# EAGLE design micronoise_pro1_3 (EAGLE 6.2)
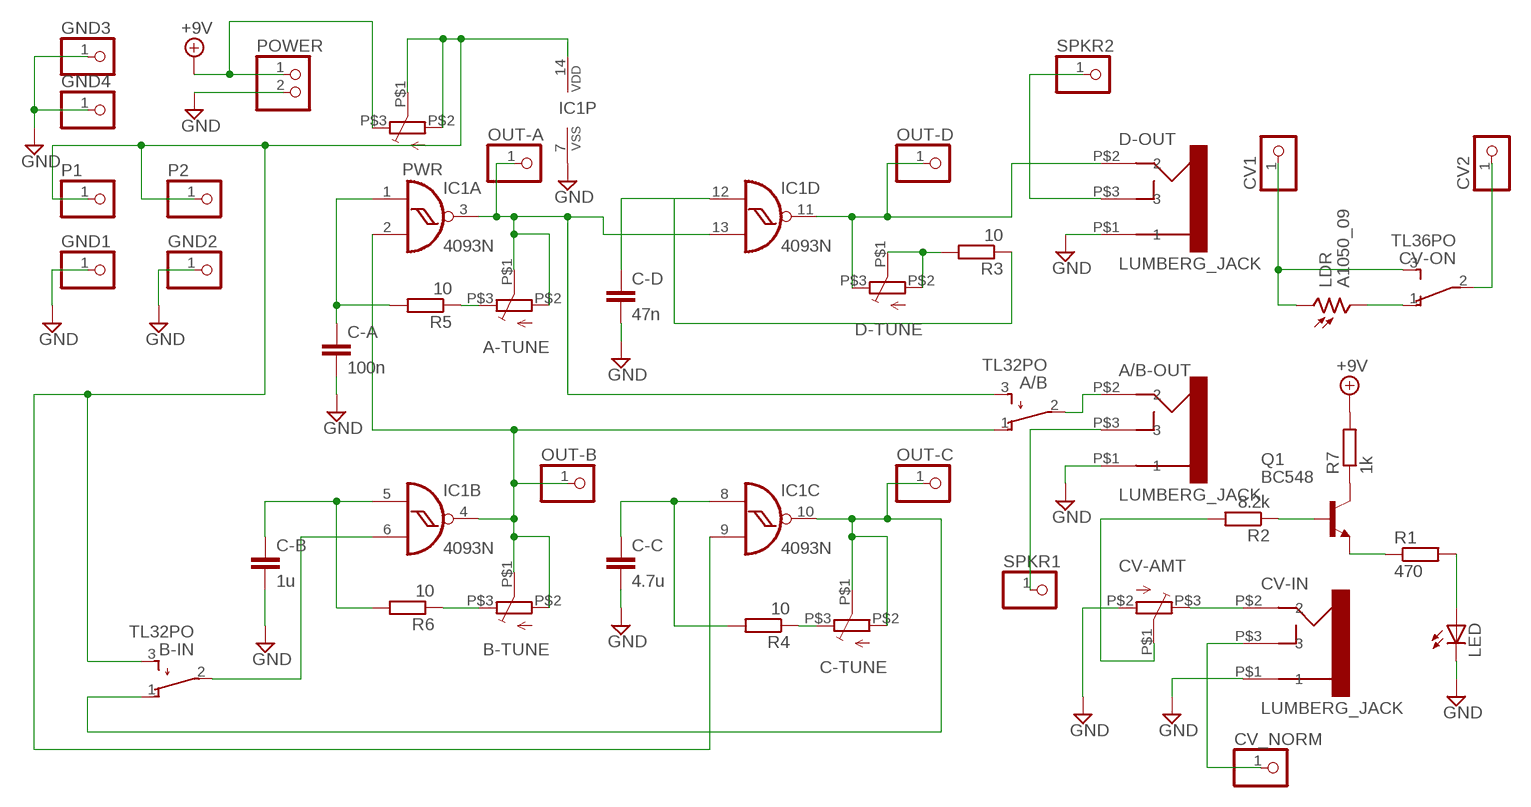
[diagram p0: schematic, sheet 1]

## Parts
A-TUNE  STR09K113  [STR09K113]
A/B  TL32PO  [TL3XPO]
A/B-OUT  LUMBERG_JACK  [JACK_CON]
B-IN  TL32PO  [TL3XPO]
B-TUNE  STR09K113  [STR09K113]
C-A  100n  C-EU050-035X075  [C050-035X075]
C-B  1u  C-EU050-035X075  [C050-035X075]
C-C  4.7u  C-EU050-035X075  [C050-035X075]
C-D  47n  C-EU050-035X075  [C050-035X075]
C-TUNE  STR09K113  [STR09K113]
CV1  PINHD-1X1  [1X01]
CV2  PINHD-1X1  [1X01]
CV-AMT  STR09K113  [STR09K113]
CV-IN  LUMBERG_JACK  [JACK_CON]
CV-ON  TL36PO  [TL3XPO]
CV_NORM  PINHD-1X1  [1X01]
D-OUT  LUMBERG_JACK  [JACK_CON]
D-TUNE  STR09K113  [STR09K113]
GND1  PINHD-1X1  [1X01]
GND2  PINHD-1X1  [1X01]
GND3  PINHD-1X1  [1X01]
GND4  PINHD-1X1  [1X01]
IC1  4093N  [DIL14]
LDR  A1050_09  [T0-46-A10XX]
LED  LED3MM  [LED3MM]
OUT-A  PINHD-1X1  [1X01]
OUT-B  PINHD-1X1  [1X01]
OUT-C  PINHD-1X1  [1X01]
OUT-D  PINHD-1X1  [1X01]
P1  PINHD-1X1  [1X01]
P2  PINHD-1X1  [1X01]
POWER  PINHD-1X2  [1X02]
PWR  STR09K113  [STR09K113]
Q1  BC548  [TO92-EBC]
R1  470  R-EU_0207/7  [0207/7]
R2  8.2k  R-EU_0207/7  [0207/7]
R3  10  R-EU_0207/7  [0207/7]
R4  10  R-EU_0207/7  [0207/7]
R5  10  R-EU_0207/7  [0207/7]
R6  10  R-EU_0207/7  [0207/7]
R7  1k  R-EU_0207/7  [0207/7]
SPKR1  PINHD-1X1  [1X01]
SPKR2  PINHD-1X1  [1X01]

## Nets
+9V: POWER.1 PWR.P$3(E) R7.2
A_TUNE: A-TUNE.P$1(W) A-TUNE.P$2(S) A/B.3(S) IC1.3(A:O) IC1.13(D:I1) OUT-A.1
GND: A/B-OUT.P$1 C-A.2 C-B.2 C-C.2 C-D.2 CV-AMT.P$2(S) CV-IN.P$1 D-OUT.P$1 GND1.1 GND2.1 GND3.1 GND4.1 IC1.7(P:VSS) LED.K(C) POWER.2
N$1: Q1.E R1.1
N$2: Q1.B R2.1
N$3: CV-ON.1(O) LDR.2
N$4: C-A.1 IC1.1(A:I0) R5.2
N$5: LED.A R1.2
N$6: CV-AMT.P$3(E) CV-IN.P$2
N$7: B-IN.3(S) IC1.9(C:I1) IC1.14(P:VDD) P1.1 P2.1 PWR.P$1(W) PWR.P$2(S)
N$8: CV2.1 CV-ON.2(P)
N$9: C-C.1 IC1.8(C:I0) R4.2
N$10: B-IN.1(O) C-TUNE.P$1(W) C-TUNE.P$2(S) IC1.10(C:O) OUT-C.1
N$11: B-IN.2(P) IC1.6(B:I1)
N$12: C-B.1 IC1.5(B:I0) R6.2
N$13: D-OUT.P$2 D-TUNE.P$3(E) IC1.11(D:O) OUT-D.1
N$14: A/B.1(O) B-TUNE.P$1(W) B-TUNE.P$2(S) IC1.2(A:I1) IC1.4(B:O) OUT-B.1
N$15: A/B-OUT.P$2 A/B.2(P)
N$16: CV1.1 CV-ON.3(S) LDR.1
N$17: CV-AMT.P$1(W) R2.2
N$18: D-OUT.P$3 SPKR2.1
N$19: A/B-OUT.P$3 SPKR1.1
N$20: CV-IN.P$3 CV_NORM.1
N$21: D-TUNE.P$1(W) D-TUNE.P$2(S) R3.2
N$22: C-TUNE.P$3(E) R4.1
N$23: A-TUNE.P$3(E) R5.1
N$24: B-TUNE.P$3(E) R6.1
N$25: C-D.1 IC1.12(D:I0) R3.1
N$26: Q1.C R7.1

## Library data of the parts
A-TUNE B-TUNE C-TUNE CV-AMT D-TUNE PWR = anyma-lib:STR09K113: Alps Potentiometer
A/B B-IN = switch:TL32PO: TINY SWITCH ON - MOM Source: http://www2.produktinfo.conrad.com/datenblaetter/700000-724999/705152-da-01-de-Subminiaturschalter_TL_36YO.pdf
A/B-OUT CV-IN D-OUT = eigene:LUMBERG_JACK: 3.5 mm Jack connector 1502 03
C-A C-B C-C C-D = rcl:C-EU: CAPACITOR, European symbol
CV1 CV2 CV_NORM GND1-GND4 OUT-A OUT-B OUT-C OUT-D P1 P2 SPKR1 SPKR2 = pinhead:PINHD-1X1: PIN HEADER
CV-ON = switch:TL36PO: TINY SWITCH ON - ON Source: http://www2.produktinfo.conrad.com/datenblaetter/700000-724999/705152-da-01-de-Subminiaturschalter_TL_36YO.pdf
IC1 = 40xx:4093: Quad 2-input NAND schmitt trigger
LDR = photo-elements:A10: Sensor Robust Light Sensing Applications
LED = led:LED: LED
POWER = pinhead:PINHD-1X2: PIN HEADER
Q1 = transistor-npn:BC548*: NPN Transistor
R1-R7 = rcl:R-EU_: RESISTOR, European symbol

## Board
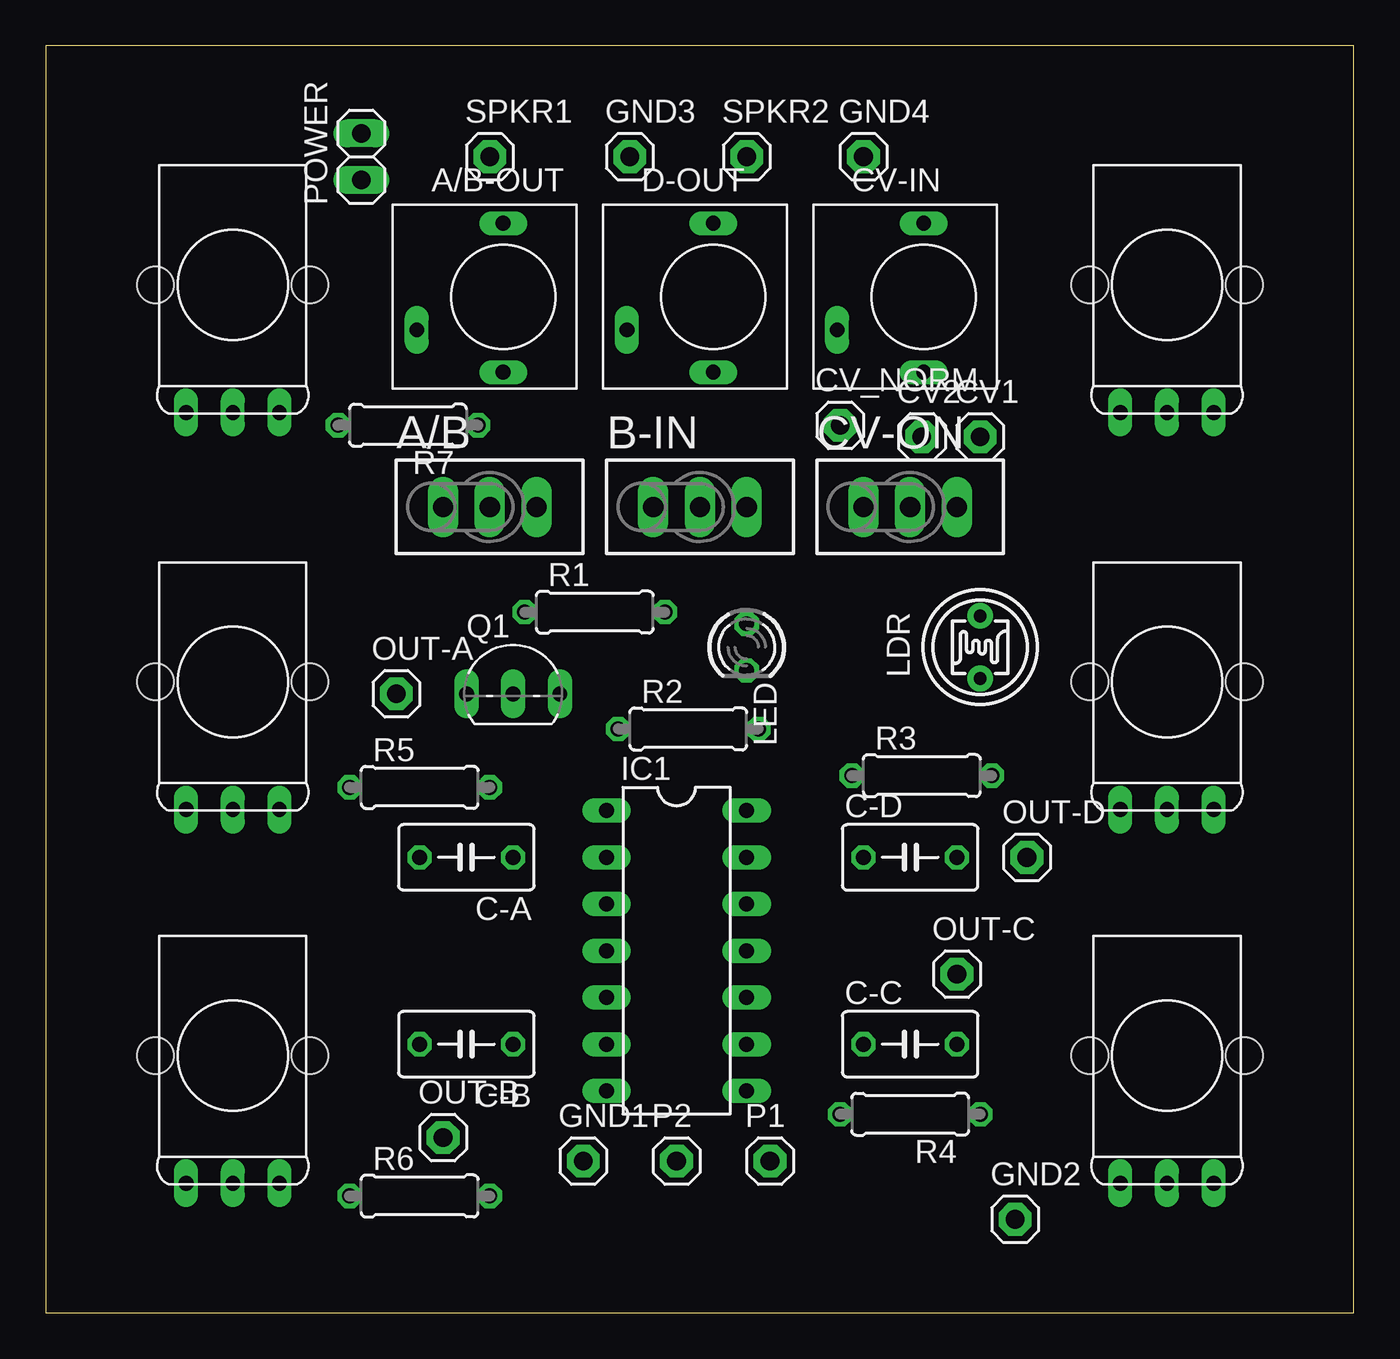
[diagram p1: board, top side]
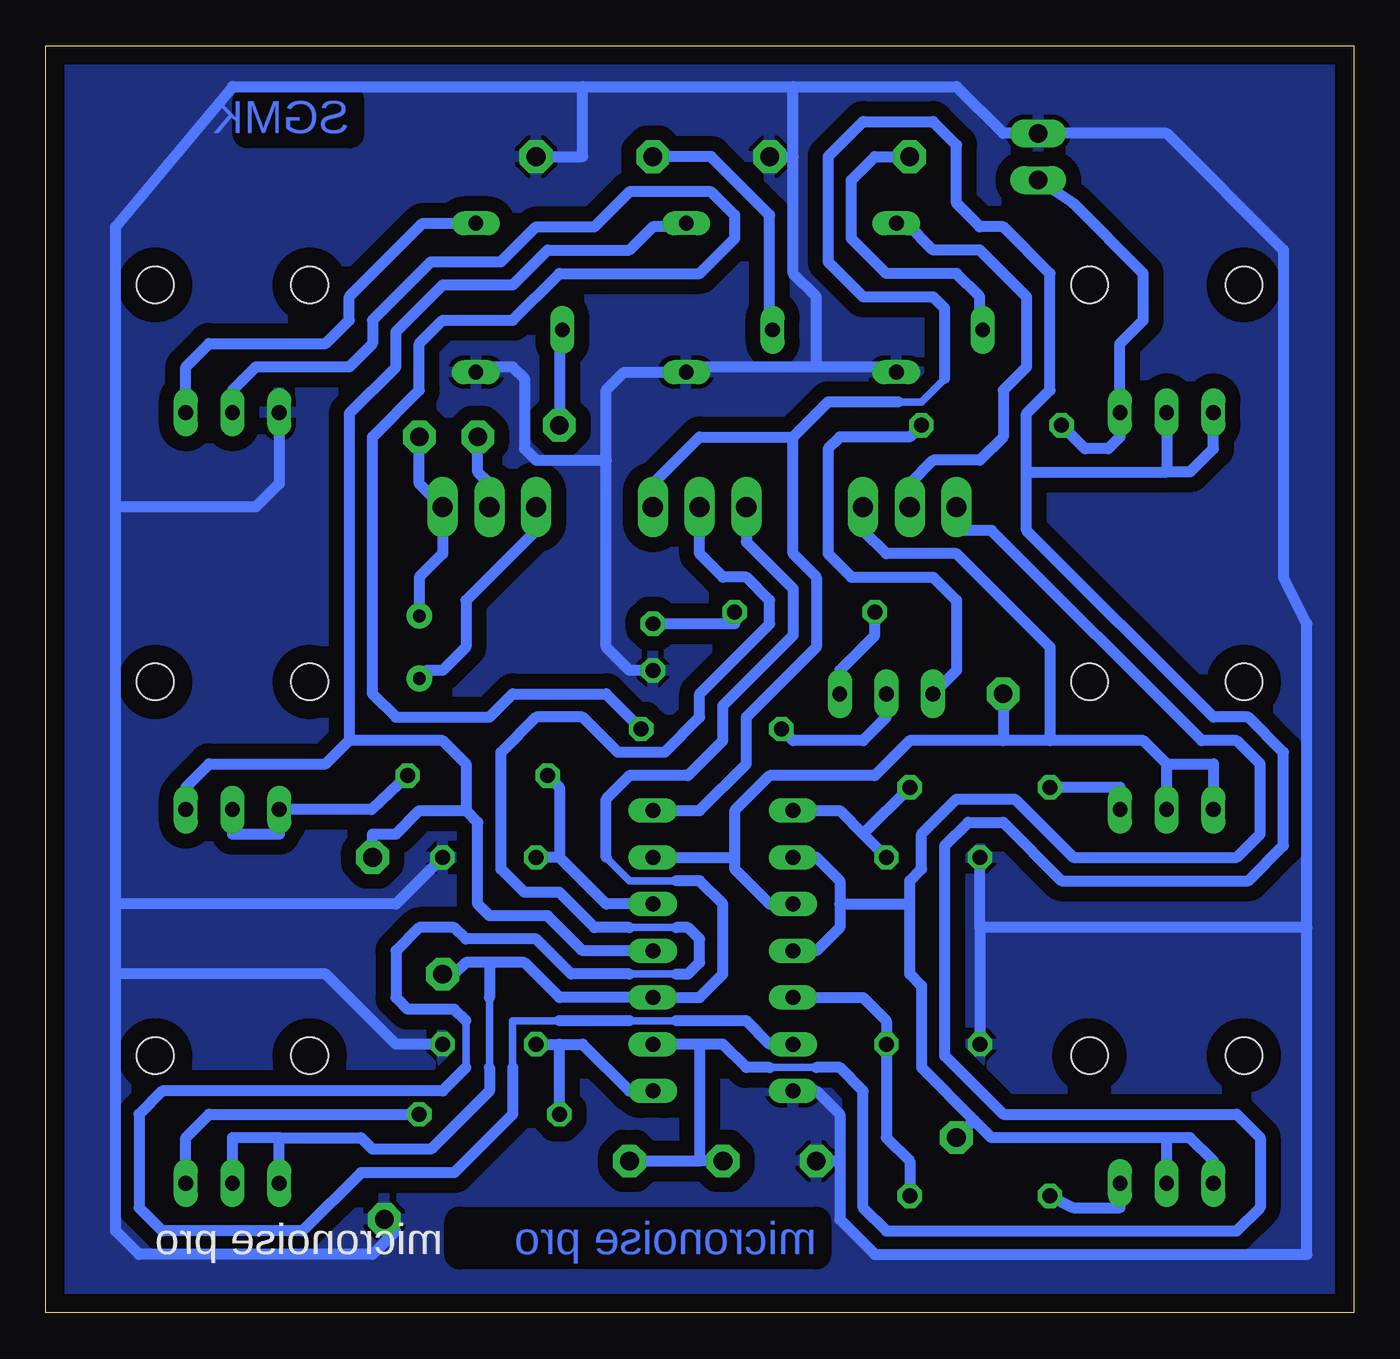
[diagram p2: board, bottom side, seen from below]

Size 71.1 x 68.89 mm. Coordinates in mm from the lower left corner, seen from the top.
Outline: 0,0 71.1,0 71.1,68.89 0,68.89 0,0
Copper layers (1*16): Top 0.035mm / dielectric 1.5mm / Bottom 0.035mm
Design rules: minimum track width 10mil, minimum drill 24mil, track to track 8mil, track to pad 8mil, pad to pad 8mil, via to via 8mil, smd to smd 8mil, copper to edge 40mil, drill to drill 8mil, minimum pad ring 10mil, minimum via ring 8mil, stop-mask expansion 4mil, vias tented up to drill 0mil, thermal gap 10mil

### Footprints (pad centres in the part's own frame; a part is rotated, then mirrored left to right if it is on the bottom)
STR09K113 = drill 0.8 long: P$1 0,0.06; P$2 -2.54,0.06; P$3 2.54,0.06 | hole 2: -4.2,7; 4.2,7
TL3XPO = drill 1.1 pad 1.422 long: 1 -2.54,0; 2 0,0; 3 2.54,0
JACK_CON = drill 0.8 long: P$1 2,-4.1; P$2 2,4; P$3 -2.7,-1.8
C050-035X075 = drill 0.813 octagon: 1 -2.54,0; 2 2.54,0
1X01 = drill 1.016 pad 1.778 octagon: 1 0,0
DIL14 = drill 0.813 long: 1 -7.62,-3.81; 2 -5.08,-3.81; 3 -2.54,-3.81; 4 0,-3.81; 5 2.54,-3.81; 6 5.08,-3.81; 7 7.62,-3.81; 8 7.62,3.81; 9 5.08,3.81; 10 2.54,3.81; 11 0,3.81; 12 -2.54,3.81; 13 -5.08,3.81; 14 -7.62,3.81
T0-46-A10XX = drill 0.7 pad 1.4: 1 -1.7,0; 2 1.7,0
LED3MM = drill 0.813 octagon: A -1.27,0; K 1.27,0
1X02 = drill 1.016 long: 1 -1.27,0; 2 1.27,0
TO92-EBC = drill 0.813 long: B 0,-1.27; C -2.54,-1.27; E 2.54,-1.27
0207/7 = drill 0.813 octagon: 1 -3.81,0; 2 3.81,0

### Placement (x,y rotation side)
A-TUNE  10.16,27.3 0 top
A/B  24.13,43.81 0 top
A/B-OUT  22.86,55.25 0 top
B-IN  35.56,43.81 0 top
B-TUNE  10.16,6.98 0 top
C-A  22.86,24.77 180 top
C-B  22.86,14.61 180 top
C-C  46.99,14.61 0 top
C-D  46.99,24.77 0 top
C-TUNE  60.96,6.98 0 top
CV1  50.8,47.62 0 top
CV2  47.62,47.62 0 top
CV-AMT  60.96,48.89 0 top
CV-IN  45.72,55.25 0 top
CV-ON  46.99,43.81 0 top
CV_NORM  43.18,48.26 0 top
D-OUT  34.29,55.25 0 top
D-TUNE  60.96,27.3 0 top
GND1  29.21,8.26 0 top
GND2  52.7,5.08 0 top
GND3  31.75,62.86 0 top
GND4  44.45,62.86 0 top
IC1  34.29,19.69 270 top
LDR  50.8,36.2 270 top
LED  38.1,36.2 270 top
OUT-A  19.05,33.66 0 top
OUT-B  21.59,9.52 0 top
OUT-C  49.53,18.41 0 top
OUT-D  53.34,24.77 0 top
P1  39.37,8.26 0 top
P2  34.29,8.26 0 top
POWER  17.14,62.86 90 top
PWR  10.16,48.89 0 top
Q1  25.4,34.92 0 top
R1  29.84,38.1 0 top
R2  34.92,31.75 0 top
R3  47.62,29.21 0 top
R4  46.99,10.8 180 top
R5  20.32,28.58 0 top
R6  20.32,6.35 0 top
R7  19.68,48.26 180 top
SPKR1  24.13,62.86 0 top
SPKR2  38.1,62.86 0 top

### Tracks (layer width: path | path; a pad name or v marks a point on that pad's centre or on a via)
+9V
  Bottom 0.61: POWER.1 15.24,60.33 11.43,56.52 11.43,53.97 12.7,52.7 PWR.P$3 12.7,47.62 13.34,46.99 14.61,46.99 R7.2
A_TUNE
  Bottom 0.61: A-TUNE.P$1 10.16,29.84 | 10.16,29.84 7.62,29.84 A-TUNE.P$2 | 10.16,29.84 11.43,31.12 16.51,31.12 | 33.66,24.77 33.66,27.3 31.75,29.21 26.03,29.21 24.13,31.12 19.05,31.12 | 33.66,24.77 33.66,24.13 31.75,22.23 IC1.3 | A/B.3 26.67,42.55 25.4,41.28 21.59,41.28 16.51,36.2 16.51,31.12 | 16.51,31.12 19.05,31.12 | IC1.13 33.66,24.77 | OUT-A.1 19.05,31.12
GND
  Bottom 0.61: 20.32,20.95 C-A.2 | 67.31,18.41 67.31,4.45 66.04,3.18 53.34,3.18 52.07,4.45 GND2.1 | 67.31,18.41 67.31,22.23 | 67.31,22.23 67.31,43.81 | 67.31,43.81 67.31,59.06 60.96,66.67 41.91,66.67 | 20.32,20.95 C-B.2 | 2.54,20.95 20.32,20.95 | A/B-OUT.P$1 25.15,51.44 29.21,51.44 | 2.54,20.95 2.54,3.18 26.03,3.18 27.94,5.08 27.94,8.26 | 2.54,20.95 2.54,37.47 3.81,40 3.81,57.78 10.16,64.14 POWER.2 19.05,64.14 21.59,66.67 30.48,66.67 | 29.21,51.44 35.56,51.44 35.85,51.14 D-OUT.P$1 39.66,51.14 40.64,50.17 40.64,46.36 | 67.31,18.41 55.88,18.41 52.07,14.61 C-C.2 | 27.94,8.26 27.94,10.8 29.21,12.06 IC1.7 | GND1.1 27.94,8.26 | 41.91,66.67 30.48,66.67 | 29.21,51.44 29.21,55.25 30.48,56.52 30.48,62.86 | 30.48,62.86 30.48,66.67 | GND3.1 30.48,62.86 | 41.91,66.67 41.91,62.86 GND4.1 | LED.K 39.37,34.92 40.64,36.2 40.64,46.36 | CV-AMT.P$2 58.42,45.09 59.69,43.81 67.31,43.81 | C-D.2 52.07,22.23 67.31,22.23 | 40.64,46.36 44.45,46.36 45.09,46.99 45.09,50.8 45.72,51.44 46.99,51.44 47.28,51.14 CV-IN.P$1
  pour Bottom (isolate 0.813): -1.27,69.22 73.66,69.22 73.66,-3.17 -1.27,-3.17
N$1
  Bottom 0.61: Q1.E 27.94,34.92 26.03,36.83 R1.1
N$2
  Bottom 0.61: Q1.B 25.4,32.38 26.67,31.12 30.48,31.12 R2.1
N$3
  Bottom 0.61: LDR.2 50.37,34.92 49.53,34.92 48.26,36.2 48.26,38.73 44.45,42.55 CV-ON.1
N$4
  Bottom 0.61: IC1.1 27.94,27.3 26.67,26.04 | 26.67,26.04 C-A.1 | R5.2 26.67,26.04
N$5
  Bottom 0.61: R1.2 33.66,37.47 LED.A
N$6
  Bottom 0.61: 47.91,59.06 CV-IN.P$2 50.61,59.25 54.61,55.25 54.61,53.97 55.88,52.7 62.23,52.7 63.5,51.44 CV-AMT.P$3 63.5,48.89
N$7
  Bottom 0.406: 31.75,13.34 29.21,13.34 | 22.22,50.8 23.49,49.53 24.77,49.53
  Bottom 0.61: 35.56,14.61 35.56,8.26 | P1.1 35.56,8.26 | P2.1 35.56,8.26 | 36.83,14.61 IC1.9 35.56,14.61 | IC1.14 35.56,27.3 33.02,29.84 33.02,32.38 29.21,36.2 29.21,40 30.48,41.28 30.48,47.62 | PWR.P$1 10.16,45.72 | 31.75,13.34 33.02,13.34 34.29,14.61 35.56,14.61 | 22.22,50.8 22.22,54.61 22.86,55.25 26.67,55.25 28.58,57.15 28.58,62.86 26.67,64.77 22.86,64.77 21.59,63.5 21.59,60.33 20.32,59.06 19.05,59.06 16.51,56.52 16.51,50.17 17.78,48.89 17.78,45.72 | 17.78,45.72 17.78,42.55 7.62,32.38 5.71,32.38 3.81,30.48 3.81,25.4 5.71,23.5 15.88,23.5 19.05,26.67 20.95,26.67 22.22,25.4 22.22,13.97 19.05,10.8 6.35,10.8 5.08,9.52 5.08,5.72 6.35,4.45 25.4,4.45 26.67,5.72 26.67,12.06 27.94,13.34 29.21,13.34 | 24.77,49.53 28.58,49.53 30.48,47.62 | 17.78,45.72 10.16,45.72 | PWR.P$2 7.62,46.99 8.89,45.72 10.16,45.72 | B-IN.3 38.1,45.09 35.56,47.62 30.48,47.62
N$8
  Bottom 0.61: CV-ON.2 46.99,45.09 47.62,45.72 CV2.1
N$9
  Bottom 0.61: C-C.1 43.18,14.61 | 43.18,14.61 41.91,14.61 39.37,12.06 IC1.8 | R4.2 43.18,14.61
N$10
  Bottom 0.406: 40.64,24.77 39.37,23.5 36.83,23.5 | 46.99,17.15 46.99,13.34
  Bottom 0.61: B-IN.1 33.02,41.91 30.48,39.37 30.48,36.83 34.29,33.02 34.29,31.12 36.2,29.21 39.37,29.21 40.64,27.94 40.64,24.77 | C-TUNE.P$1 60.96,9.52 58.42,9.52 | C-TUNE.P$2 58.42,9.52 | 58.42,9.52 53.98,9.52 53.34,8.89 50.16,8.89 46.99,12.06 46.99,13.34 | 36.83,23.5 35.56,23.5 34.29,22.23 34.29,18.41 35.56,17.15 IC1.10 43.18,17.15 45.09,19.05 46.99,19.05 | 46.99,19.05 48.26,19.05 48.89,18.41 OUT-C.1 | 46.99,19.05 46.99,17.15
N$11
  Bottom 0.406: 39.37,18.41 36.83,18.41 | 36.83,20.95 39.37,20.95 | 36.83,15.88 39.37,15.88 | 43.18,15.88 45.72,15.88 45.72,13.34 | 48.26,15.88 48.26,13.34
  Bottom 0.61: IC1.6 31.75,14.61 33.02,15.88 36.83,15.88 | 48.26,13.34 49.53,12.06 64.77,12.06 66.04,10.8 66.04,5.72 64.77,4.45 57.15,4.45 53.98,7.62 48.89,7.62 45.72,10.8 45.72,13.34 | 36.83,18.41 36.2,18.41 35.56,19.05 35.56,20.32 36.2,20.95 36.83,20.95 | 39.37,20.95 41.27,20.95 43.18,22.86 45.09,22.86 46.35,24.13 46.35,30.48 44.45,32.38 41.91,32.38 40.01,30.48 37.46,30.48 35.56,32.38 35.56,33.66 31.75,37.47 31.75,38.73 33.02,40 34.29,40 35.56,41.28 B-IN.2 | 39.37,18.41 42.55,18.41 44.45,20.32 48.26,20.32 48.89,20.95 50.8,20.95 52.07,19.69 52.07,17.15 51.44,16.51 48.89,16.51 48.26,15.88 | 39.37,15.88 43.18,15.88
N$12
  Bottom 0.61: IC1.5 26.67,17.15 25.4,15.88 C-B.1 25.4,9.52 24.13,8.26 R6.2
N$13
  Bottom 0.61: D-OUT.P$2 36.48,59.06 38.1,59.06 39.37,57.78 43.81,57.78 45.72,55.88 49.53,55.88 52.07,53.34 52.07,51.44 54.61,48.89 54.61,31.12 | IC1.11 41.91,19.69 43.81,21.59 46.99,21.59 47.62,22.23 47.62,26.67 48.26,27.3 | OUT-D.1 53.34,26.04 52.07,26.04 50.8,27.3 48.26,27.3 | 54.61,31.12 55.88,29.84 62.23,29.84 63.5,28.58 D-TUNE.P$3 | 54.61,31.12 49.53,31.12 48.26,29.84 48.26,27.3
N$14
  Bottom 0.61: IC1.2 29.21,24.77 27.94,23.5 27.94,22.23 | 20.64,10.48 23.49,13.34 23.49,17.78 24.13,18.41 24.13,22.23 | 20.64,10.48 19.68,9.52 10.16,9.52 | 24.13,22.23 24.13,23.5 23.49,24.13 23.49,26.04 21.59,27.94 18.41,27.94 15.24,24.77 6.35,24.77 5.08,26.04 5.08,29.84 6.35,31.12 8.25,31.12 19.68,42.55 21.59,42.55 A/B.1 | IC1.4 29.21,19.69 27.94,20.95 27.94,22.23 | B-TUNE.P$2 7.62,8.26 8.89,9.52 10.16,9.52 | B-TUNE.P$1 10.16,9.52 | 27.94,22.23 24.13,22.23 | OUT-B.1 20.64,10.48
N$15
  Bottom 0.61: A/B.2 24.13,45.09 22.86,46.36 20.32,46.36 19.05,47.62 19.05,50.17 17.78,51.44 17.78,55.25 20.32,57.78 22.86,57.78 24.32,59.25 A/B-OUT.P$2
N$16
  Bottom 0.61: CV1.1 50.8,45.09 CV-ON.3 49.53,41.28 50.8,40 LDR.1
N$17
  Bottom 0.61: 60.96,48.89 CV-AMT.P$1 60.96,50.17 59.69,51.44 54.61,51.44 53.34,52.7 53.34,53.97 50.16,57.15 46.35,57.15 44.45,59.06 41.27,59.06 39.37,60.96 34.92,60.96 33.66,59.69 33.66,58.42 35.56,56.52 43.18,56.52 45.72,53.97 49.53,53.97 50.8,52.7 50.8,50.17 53.34,47.62 53.34,33.66 52.07,32.38 46.99,32.38 45.72,33.66 40.64,33.66 R2.2
N$18
  Bottom 0.61: D-OUT.P$3 31.75,53.61 31.75,59.69 34.92,62.86 SPKR2.1
N$19
  Bottom 0.61: A/B-OUT.P$3 20.32,53.61 20.32,55.25 21.59,56.52 25.4,56.52 27.3,58.42 27.3,61.59 26.03,62.86 SPKR1.1
N$20
  Bottom 0.61: CV-IN.P$3 43.18,53.45 CV_NORM.1
N$21
  Bottom 0.61: R3.2 53.4,27.37 D-TUNE.P$2 58.42,26.04 60.96,26.04 D-TUNE.P$1
N$22
  Bottom 0.61: C-TUNE.P$3 63.5,9.52 62.23,10.8 R4.1
N$23
  Bottom 0.61: A-TUNE.P$3 12.7,28.58 R5.1
N$24
  Bottom 0.61: R6.1 15.24,5.72 12.7,5.72 B-TUNE.P$3
N$25
  Bottom 0.61: IC1.12 40.64,22.23 43.18,24.77 | 43.18,24.77 C-D.1 | R3.1 43.18,28.58 43.18,24.77
N$26
  Bottom 0.61: R7.1 24.13,47.62 27.94,47.62 28.58,46.99 28.58,41.28 27.3,40 22.86,40 21.59,38.73 21.59,34.92 Q1.C

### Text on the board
Bottom: SGMK | micronoise pro
bNames: micronoise pro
